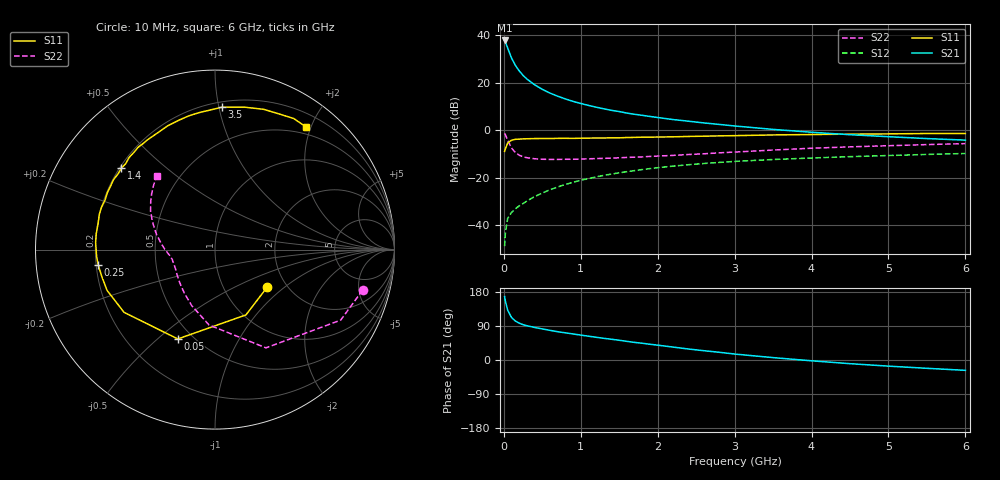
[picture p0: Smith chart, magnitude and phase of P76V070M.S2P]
! SIEMENS Small Signal Semiconductors
! BFP196
! Si NPN RF Bipolar Junction Transistor in SOT143
! VCE = 6 V  IC = 70 mA
! Common Emitter S-Parameters:  May  1996
# GHz  S  MA  R  50
!  f  S11  S21  S12  S22
! GHz  MAG  ANG  MAG  ANG  MAG  ANG  MAG  ANG
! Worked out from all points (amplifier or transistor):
!   36 points, 10 MHz to 6 GHz, reference 50 ohm
!   highest |S21| = 37.8 dB at 10 MHz (marker M1)
!   |S21| within 3 dB of that: start of sweep to 47.35 MHz
!   unconditionally stable (mu >= 1): 435.6 MHz to 4.465 GHz
!   at 250 MHz: K = 0.87, MSG = 27.0 dB, |S12| = -30.9 dB
!   at 1.4 GHz: K = 1.09, MAG = 11.6 dB, |S12| = -18.5 dB
!   at 6 GHz: K = 0.98, MSG = 2.8 dB, |S12| = -9.8 dB
!   S11 on the Smith chart (normalised r, x): 10 MHz: 1.60, -0.76; 50 MHz: 0.42, -0.58; 250 MHz: 0.21, -0.06; 1.4 GHz: 0.21, +0.36; 3.5 GHz: 0.24, +1.02; 6 GHz: 0.39, +1.92
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0.01  0.3581 -35.6  77.85 167.5  0.0036 76.8  0.8532 -15.3
0.02  0.4026 -64.6  71.95 155.5  0.0068 71.2  0.8029 -29.3
0.05  0.5391 -112.6  53.71 131.4  0.0139 55.9  0.6166 -62.6
0.1  0.6156 -145.4  33.17 112.1  0.0185 48.0  0.4215 -94.5
0.15  0.6428 -159.3  23.24 102.8  0.0221 50.3  0.3375 -112.7
0.2  0.6485 -166.8  17.79 97.2  0.0255 53.5  0.2973 -124.9
0.25  0.6561 -172.4  14.28 93.3  0.0285 56.2  0.2749 -134.0
0.3  0.6606 -176.6  11.98 90.4  0.0322 57.4  0.2636 -140.1
0.4  0.6662 176.6  9.066 85.9  0.0399 61.0  0.2501 -149.2
0.5  0.6677 172.2  7.262 82.0  0.0474 62.6  0.2441 -154.9
0.6  0.6671 167.4  6.05 78.3  0.0556 62.9  0.2426 -159.2
0.7  0.6738 163.0  5.206 74.6  0.0636 63.4  0.2425 -162.1
0.9  0.6719 155.7  4.047 68.7  0.0801 62.2  0.2441 -166.9
1.1  0.6806 148.8  3.331 62.8  0.0956 60.4  0.2498 -170.0
1.4  0.6918 138.9  2.619 54.7  0.119 56.7  0.2581 -173.9
1.7  0.7055 129.7  2.164 46.4  0.1408 52.5  0.2705 -178.3
2.2  0.725 116.0  1.677 34.1  0.1751 45.0  0.2948 175.3
3  0.7679 96.8  1.228 15.7  0.2199 33.1  0.3463 163.2
3.5  0.7947 87.1  1.041 6.3  0.2413 26.1  0.3819 155.9
4.5  0.8272 70.9  0.804 -9.7  0.2771 14.2  0.4457 143.5
5.5  0.852 59.0  0.666 -21.9  0.3087 3.5  0.4976 133.3
6  0.851 53.5  0.618 -27.3  0.323 -2.1  0.5213 128.4
